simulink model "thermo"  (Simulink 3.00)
settings: Solver=ode45  SolverMode=SingleTasking  StartTime=0.0  StopTime=2*24*60*60  FixedStep=100  RelTol=1e-3  AbsTol=1e-6
PreLoadFcn:
  | thermdat
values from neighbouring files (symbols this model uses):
  c = c .* (cnz+repmat(zeroc,[p n]))    [rss.m]    (also in thermdat.m = 1005.4)
  cost = 0.09/3.6e6    (= 2.5e-08)    [thermdat.m]
  ha = THeater*c    (= 304636.2)    [thermdat.m]
  M = (lenHouse*widHouse*htHouse+tan(pitRoof)*widHouse*lenHouse)*densAir    [thermdat.m]
  Mdot = 0.1    [thermdat.m]
  Req = RWall*RWindow/(RWall + RWindow)    [thermdat.m]
  TinIC = 20    [thermdat.m]
libraries: simulink_extras x3

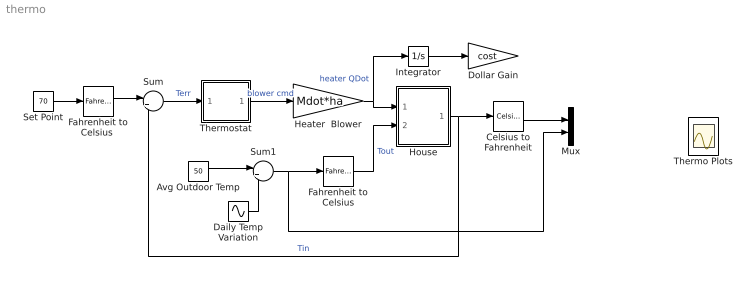
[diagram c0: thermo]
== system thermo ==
  Avg Outdoor Temp : Constant  Value=50
  Celsius to Fahrenheit : simulink_extras/Transformations/Celsius to Fahrenheit
  Daily Temp Variation : Sin  Amplitude=15  Frequency=2*pi/(24*3600)  Phase=0  SampleTime=0
  Dollar Gain : Gain  Gain=cost  SaturateOnIntegerOverflow=on
  Fahrenheit to Celsius : simulink_extras/Transformations/Fahrenheit to Celsius
  "Fahrenheit to Celsius " : simulink_extras/Transformations/Fahrenheit to Celsius
  Heater  Blower : Gain  Gain=Mdot*ha  SaturateOnIntegerOverflow=on
  House : Subsystem
  Integrator : Integrator  ExternalReset=none  InitialConditionSource=internal  InitialCondition=0  LimitOutput=off  UpperSaturationLimit=inf  LowerSaturationLimit=-inf  ShowSaturationPort=off  ShowStatePort=off  AbsoluteTolerance=auto
  Mux : Mux  Inputs=2
  Set Point : Constant  Value=70
  Sum : Sum  Inputs=|+-  SaturateOnIntegerOverflow=on
  Sum1 : Sum  Inputs=|++  SaturateOnIntegerOverflow=on
  Thermo Plots : Scope  NumInputPorts=2
  Thermostat : Subsystem
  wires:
  Set Point/1 -> "Fahrenheit to Celsius "/1
  "Fahrenheit to Celsius "/1 -> Sum/1
  Integrator/1 -> Dollar Gain/1
  Heater  Blower/1 -> Integrator/1, House/1(Heater QDot In)  "heater QDot"
  Thermostat/1(Blower switch) -> Heater  Blower/1  "blower cmd"
  Sum/1 -> Thermostat/1(Terr)  "Terr"
  House/1(Indoor Temp Tin) -> Sum/2, Celsius to Fahrenheit/1  "Tin"
  Daily Temp Variation/1 -> Sum1/2
  Sum1/1 -> Fahrenheit to Celsius/1, Mux/2
  Avg Outdoor Temp/1 -> Sum1/1
  Celsius to Fahrenheit/1 -> Mux/1
  Fahrenheit to Celsius/1 -> House/2(Outdoor Temp Tout)  "Tout"
  ? -> ?  "Indoor vs. Outd]\r \t  Position\t\t  [85, 15, 105, 35]\r \t  TriggerType"
  ?In/1 -> ?Out/1

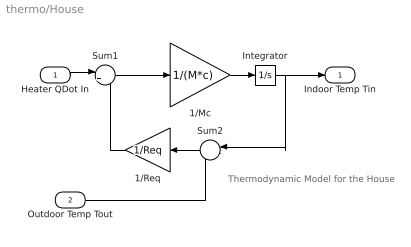
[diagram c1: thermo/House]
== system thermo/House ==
  note: Thermodynamic Model for the House
  Heater QDot In : Inport  Port=1  PortWidth=-1  SampleTime=-1  DataType=auto
  Outdoor Temp Tout : Inport  Port=2  PortWidth=-1  SampleTime=-1  DataType=auto
  1/Mc : Gain  Gain=1/(M*c)  SaturateOnIntegerOverflow=on
  1/Req : Gain  Orientation=left  Gain=1/Req  SaturateOnIntegerOverflow=on
  Integrator : Integrator  ExternalReset=none  InitialConditionSource=internal  InitialCondition=TinIC  LimitOutput=off  UpperSaturationLimit=inf  LowerSaturationLimit=-inf  ShowSaturationPort=off  ShowStatePort=off  AbsoluteTolerance=auto
  Sum1 : Sum  Inputs=|++  SaturateOnIntegerOverflow=on
  Sum2 : Sum  Orientation=left  Inputs=|-+  SaturateOnIntegerOverflow=on
  Indoor Temp Tin : Outport  Port=1  InitialOutput=0
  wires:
  Outdoor Temp Tout/1 -> Sum2/2
  Heater QDot In/1 -> Sum1/1
  Sum1/1 -> 1/Mc/1
  Sum2/1 -> 1/Req/1
  1/Req/1 -> Sum1/2
  1/Mc/1 -> Integrator/1
  Integrator/1 -> Sum2/1, Indoor Temp Tin/1

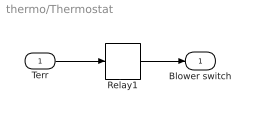
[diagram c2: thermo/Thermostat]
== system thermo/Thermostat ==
  Terr : Inport  Port=1  PortWidth=-1  SampleTime=-1  DataType=auto
  Relay1 : Relay  OnSwitchValue=5*(5/9)  OffSwitchValue=-5*(5/9)  OnOutputValue=1  OffOutputValue=0
  Blower switch : Outport  Port=1  InitialOutput=0
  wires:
  Terr/1 -> Relay1/1
  Relay1/1 -> Blower switch/1
